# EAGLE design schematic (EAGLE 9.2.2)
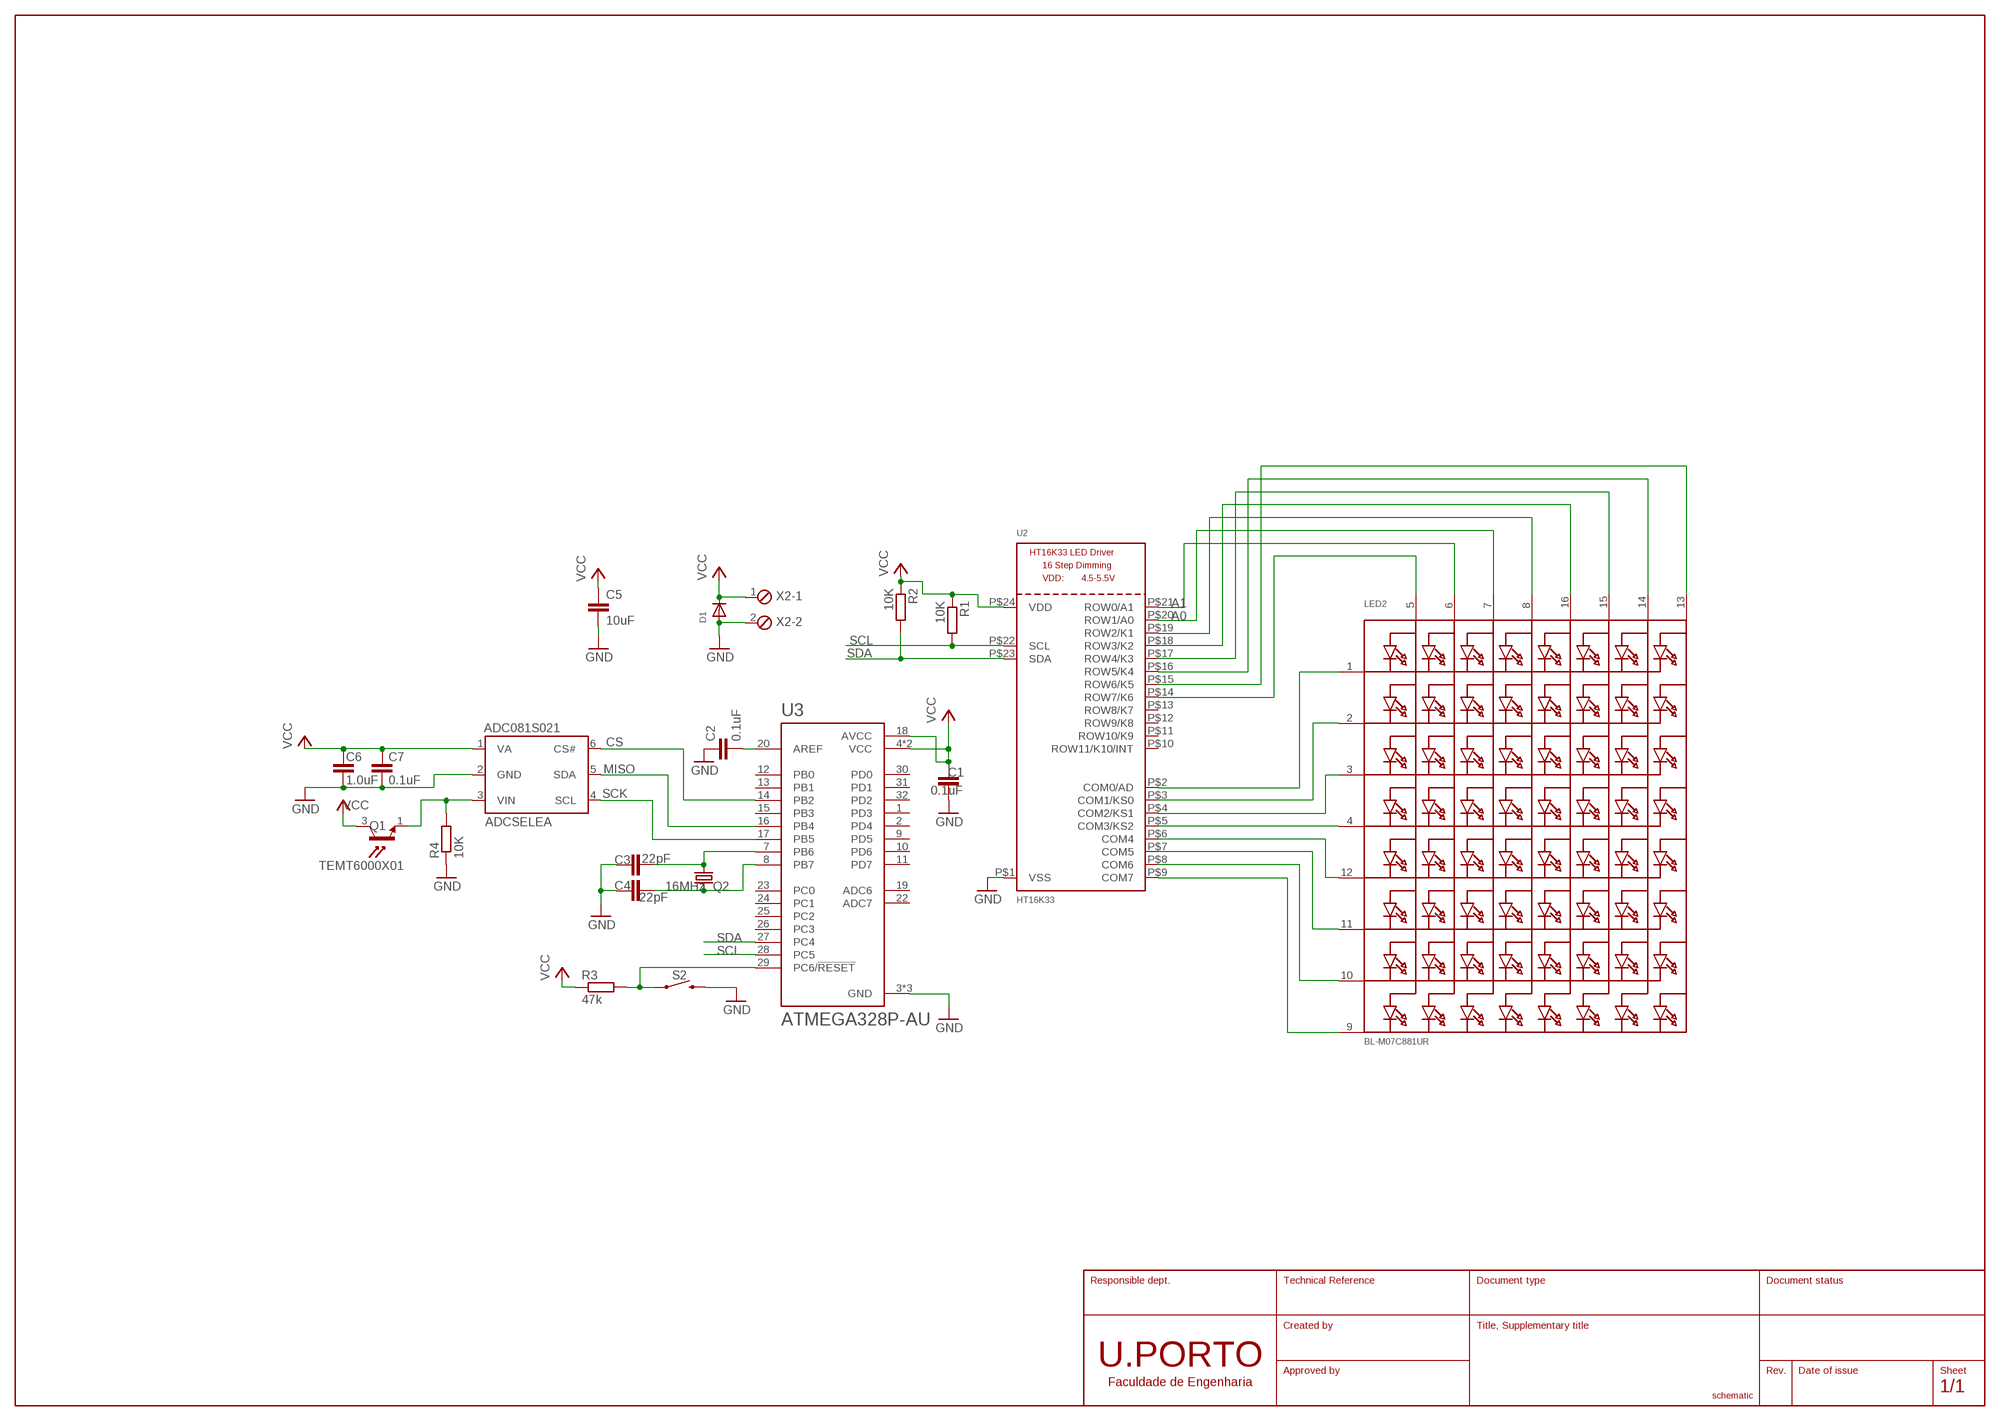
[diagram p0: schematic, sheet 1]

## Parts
ADC081S021  ADCSELEA  [SOT23]
C1  0.1uF  0.1UF-0402-16V-10%  [0402]
C2  0.1uF  0.1UF-0402-16V-10%  [0402]
C3  22pF  22PF-0603-50V-5%  [0603]
C4  22pF  22PF-0603-50V-5%  [0603]
C5  10uF  10UF-0603-6.3V-20%  [0603]
C6  1.0uF  1.0UF-0402-16V-10%  [0402]
C7  0.1uF  0.1UF-0402-16V-10%  [0402]
D1  DIODESOD-323F  [SOD-323F]
LED2  BL-M07C881UR  DISP_SEGMENT_8X8_ROWCATHODE  [SEGMENT_BL-M07C881UR]
Q1  TEMT6000X01  [TRANS_TEMT6000X01]
Q2  16MHz  CRYSTALCTS406  [CTS406]
R1  10K  R-EU_M0805  [M0805]
R2  10K  R-EU_M0805  [M0805]
R3  47k  R-EU_M0805  [M0805]
R4  10K  R-EU_M0805  [M0805]
S2  MOMENTARY-SWITCH-SPST-SMD-6.0X3.5MM  [TACTILE_SWITCH_SMD_6.0X3.5MM]
U2  HT16K33  HT16K33_SOP24  [SOP24_300MIL]
U3  ATMEGA328P-AU  [QFP80P900X900X120-32N]
X2  MPT2  [2POL254]

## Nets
A0 [LEDS]: LED2.7(A3) U2.P$20(ROW1/A0)
A1 [LEDS]: LED2.6(A2) U2.P$21(ROW0/A1)
CS [OTHER]: ADC081S021.6(CS#) U3.14(PB2)
GND [GND]: ADC081S021.2(GND) C1.1 C2.1 C3.1 C4.1 C5.2 C6.2 C7.2 D1.A R4.1 S2.2 U2.P$1(VSS) U3.3(GND) U3.5(GND) U3.21(GND) X2.2
MISO [OTHER]: ADC081S021.5(SDA) U3.16(PB4)
N$1 [OTHER]: C3.2 Q2.1 U3.7(PB6)
N$2 [OTHER]: C4.2 Q2.3 U3.8(PB7)
N$3 [OTHER]: C2.2 U3.20(AREF)
N$6 [LEDS]: LED2.9(K8) U2.P$9(COM7)
N$7 [LEDS]: LED2.10(K7) U2.P$8(COM6)
N$8 [LEDS]: LED2.11(K6) U2.P$7(COM5)
N$9 [LEDS]: LED2.12(K5) U2.P$6(COM4)
N$10 [LEDS]: LED2.4(K4) U2.P$5(COM3/KS2)
N$11 [LEDS]: LED2.3(K3) U2.P$4(COM2/KS1)
N$12 [LEDS]: LED2.2(K2) U2.P$3(COM1/KS0)
N$13 [LEDS]: LED2.1(K1) U2.P$2(COM0/AD)
N$14 [LEDS]: LED2.8(A4) U2.P$19(ROW2/K1)
N$15 [LEDS]: LED2.16(A5) U2.P$18(ROW3/K2)
N$16 [LEDS]: LED2.15(A6) U2.P$17(ROW4/K3)
N$17 [OTHER]: ADC081S021.3(VIN) Q1.1(E) R4.2
N$19 [LEDS]: LED2.5(A1) U2.P$14(ROW7/K6)
N$34 [OTHER]: R3.2 S2.1 U3.29(PC6/!RESET)
SCK [OTHER]: ADC081S021.4(SCL) U3.17(PB5)
SCL [OTHER]: R1.2 U2.P$22(SCL) U3.28(PC5)
SDA [OTHER]: R2.2 U2.P$23(SDA) U3.27(PC4)
SEG_F [LEDS]: LED2.14(A7) U2.P$16(ROW5/K4)
SEG_G [LEDS]: LED2.13(A8) U2.P$15(ROW6/K5)
VCC: ADC081S021.1(VA) C1.2 C5.1 C6.1 C7.1 D1.C Q1.3(C) R1.1 R2.1 R3.1 U2.P$24(VDD) U3.4(VCC) U3.6(VCC) U3.18(AVCC) X2.1
Unconnected: U2.P$10(ROW11/K10/INT) U2.P$11(ROW10/K9) U2.P$12(ROW9/K8) U2.P$13(ROW8/K7) U3.1(PD3) U3.2(PD4) U3.9(PD5) U3.10(PD6) U3.11(PD7) U3.12(PB0) U3.13(PB1) U3.15(PB3) U3.19(ADC6) U3.22(ADC7) U3.23(PC0) U3.24(PC1) U3.25(PC2) U3.26(PC3) U3.30(PD0) U3.31(PD1) U3.32(PD2)

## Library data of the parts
ADC081S021 = pmodals:ADCSELE
C1 C2 C7 = SparkFun-Capacitors:0.1UF: 0.1µF ceramic capacitors; PROD_ID: CAP-12416
C3 C4 = SparkFun-Capacitors:22PF: 22pF ceramic capacitors; PROD_ID: CAP-07876
C5 = SparkFun-Capacitors:10UF: 10.0µF ceramic capacitors; PROD_ID: CAP-11015
C6 = SparkFun-Capacitors:1.0UF: 1µF ceramic capacitors; PROD_ID: CAP-12417
D1 = adafruit:DIODE: Diode
LED2 = microbuilder:DISP_SEGMENT_8X8_ROWCATHODE: 8x8 LED Segment Displays: Row = Cathode 0.7" Red 8X8 Matrix, 1.9mm Round LEDs - BL-M07C881UR 1.2" Red 8x8 Matrix, 3.0mm Round LEDs - BL-M12A881UR 1.2" Red 8x8 Matrix, 3.0mm Square LEDs - BL-M12A883
Q1 = TEMT6000X01:TEMT6000X01: Ambient Light Sensor Phototransistor Chip Silicon 570nm Automotive 3-Pin SMD T/R; AVAILABILITY: Unavailable; DESCRIPTION: Ambient Light Sensor Phototransistor Chip Silicon 570nm Automotive 3-Pin SMD T/R; MF: Vishay Semiconductor; MP: TEMT6000X01; PACKAGE: 1206 Vishay; PRICE: None
Q2 = adafruit:CRYSTAL: CRYSTAL; OC_FARNELL: unknown; OC_NEWARK: unknown
R1-R4 = rcl:R-EU_: RESISTOR, European symbol; SPICEPREFIX: R
S2 = SparkFun-Switches:MOMENTARY-SWITCH-SPST: Momentary Switch (Pushbutton) - SPST; PROD_ID: SWCH-00815; SF_SKU: COM-08229
U2 = microbuilder:HT16K33_SOP24
U3 = ATMEGA328P-AU:ATMEGA328P-AU: ATmega Series 20 MHz 32 KB Flash 2 KB SRAM 8-Bit Microcontroller - TQFP-32; AVAILABILITY: Unavailable; DESCRIPTION: Microcontroller Mcu, 8 Bit, Atmega, 20mhz, Tqfp-32; MF: Microchip; MP: ATMEGA328P-AU; PACKAGE: TQFP-32 Microchip; PRICE: None
X2 = con-phoenix-254:MPT2: PHOENIX CONNECTOR; OC_FARNELL: unknown; OC_NEWARK: unknown

## Module ADC081S021
Ports: SDA(io) SCL(io) CS#(io) VA(io) GND(io) VIN(io)

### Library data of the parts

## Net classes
0 VCC: width 0.254 mm, clearance 0.203 mm
1 GND: width 0.254 mm, clearance 0.203 mm
2 OTHER: width 0.254 mm, clearance 0.203 mm
3 LEDS: width 0.254 mm, clearance 0.203 mm

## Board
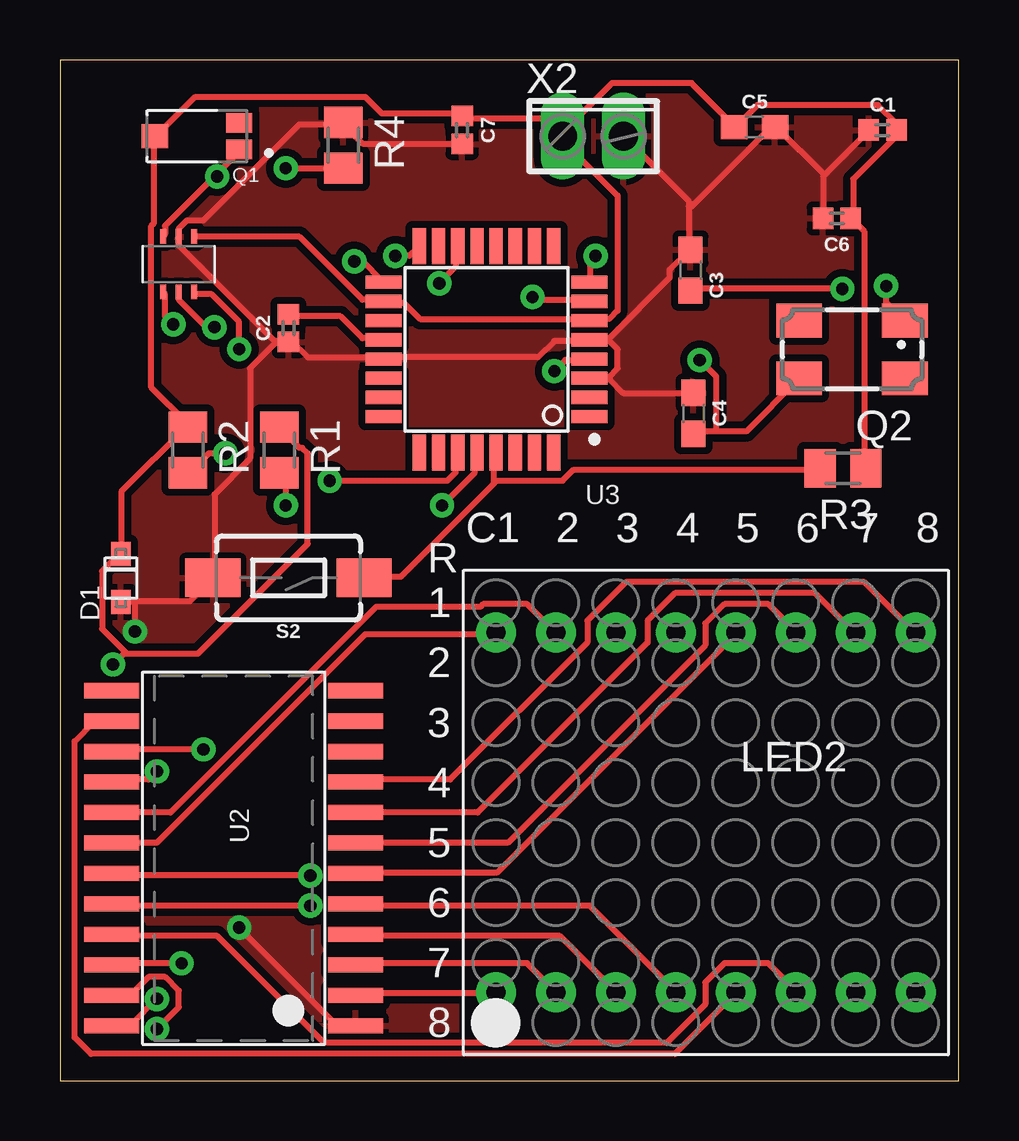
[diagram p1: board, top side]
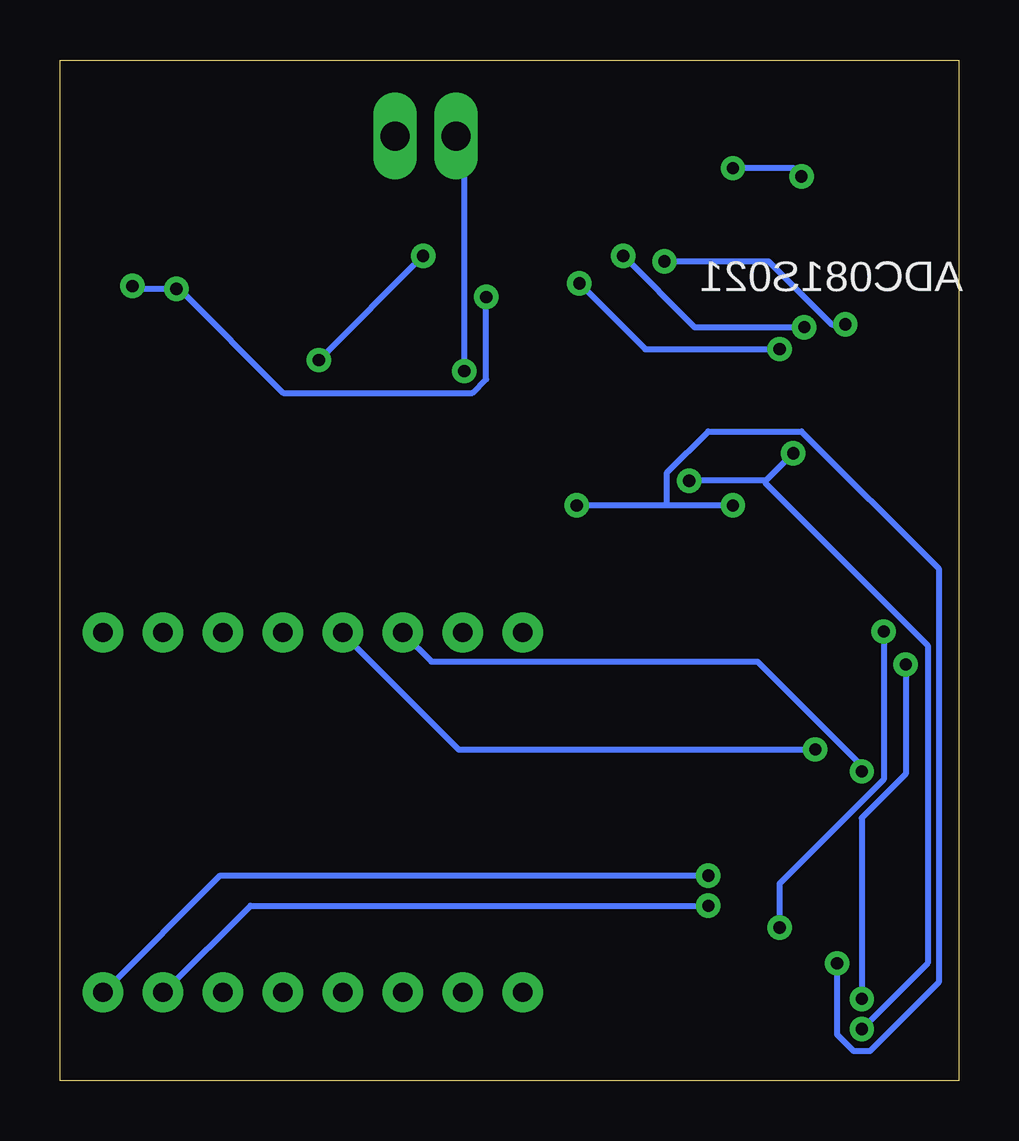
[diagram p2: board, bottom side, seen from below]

Size 37.47 x 42.55 mm. Coordinates in mm from the lower left corner, seen from the top.
Outline: 0,0 37.47,0 37.47,42.55 0,42.55 0,0
Copper layers (1*16): Top 0.035mm / dielectric 1.5mm / Bottom 0.035mm
Design rules "SparkFun": minimum track width 8mil, minimum drill 20mil, track to track 8mil, track to pad 8mil, pad to pad 8mil, via to via 8mil, smd to smd 8mil, copper to edge 10mil, drill to drill 8mil, minimum pad ring 12mil, minimum via ring 10mil, stop-mask expansion 4mil, vias tented up to drill 25mil, thermal gap 10mil

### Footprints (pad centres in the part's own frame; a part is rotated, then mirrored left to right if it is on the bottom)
SOT23 = smd 0.25 x 0.6: 1 -0.65,-1.15; 2 0,-1.15; 3 0.65,-1.15; 4 0.65,1.15; 5 0,1.15; 6 -0.65,1.15
0402 = smd 0.85 x 0.9: 1 -0.58,0; 2 0.58,0
0603 = smd 1.1 x 1: 1 -0.85,0; 2 0.85,0
SOD-323F = smd 1 x 0.8: A -1,0; C 1,0
SEGMENT_BL-M07C881UR = drill 0.8 pad 1.676: 1 -8.75,-7.5; 2 -6.25,-7.5; 3 -3.75,-7.5; 4 -1.25,-7.5; 5 1.25,-7.5; 6 3.75,-7.5; 7 6.25,-7.5; 8 8.75,-7.5; 9 8.75,7.5; 10 6.25,7.5; 11 3.75,7.5; 12 1.25,7.5; 13 -1.25,7.5; 14 -3.75,7.5; 15 -6.25,7.5; 16 -8.75,7.5
TRANS_TEMT6000X01 = smd 1.1 x 0.8: 1 -1.755,0.55; 2 -1.755,-0.55 | smd 1.1 x 1: 3 1.755,0
CTS406 = smd 1.9 x 1.4: 1 -2.2,-1.2; 2 2.2,-1.2; 3 2.2,1.2; 4 -2.2,1.2
M0805 = smd 1.3 x 1.6: 1 -0.95,0; 2 0.95,0
TACTILE_SWITCH_SMD_6.0X3.5MM = smd 2.3 x 1.6: 1 -3.15,0; 2 3.15,0
SOP24_300MIL = smd 0.635 x 2.286: P$1 -6.985,-5.08; P$2 -5.715,-5.08; P$3 -4.445,-5.08; P$4 -3.175,-5.08; P$5 -1.905,-5.08; P$6 -0.635,-5.08; P$7 0.635,-5.08; P$8 1.905,-5.08; P$9 3.175,-5.08; P$10 4.445,-5.08; P$11 5.715,-5.08; P$12 6.985,-5.08; P$13 6.985,5.08; P$14 5.715,5.08; P$15 4.445,5.08; P$16 3.175,5.08; P$17 1.905,5.08; P$18 0.635,5.08; P$19 -0.635,5.08; P$20 -1.905,5.08; P$21 -3.175,5.08; P$22 -4.445,5.08; P$23 -5.715,5.08; P$24 -6.985,5.08
QFP80P900X900X120-32N = smd 1.5 x 0.55: 1 -4.3,2.8; 2 -4.3,2; 3 -4.3,1.2; 4 -4.3,0.4; 5 -4.3,-0.4; 6 -4.3,-1.2; 7 -4.3,-2; 8 -4.3,-2.8; 17 4.3,-2.8; 18 4.3,-2; 19 4.3,-1.2; 20 4.3,-0.4; 21 4.3,0.4; 22 4.3,1.2; 23 4.3,2; 24 4.3,2.8 | smd 0.55 x 1.5: 9 -2.8,-4.3; 10 -2,-4.3; 11 -1.2,-4.3; 12 -0.4,-4.3; 13 0.4,-4.3; 14 1.2,-4.3; 15 2,-4.3; 16 2.8,-4.3; 25 2.8,4.3; 26 2,4.3; 27 1.2,4.3; 28 0.4,4.3; 29 -0.4,4.3; 30 -1.2,4.3; 31 -2,4.3; 32 -2.8,4.3
2POL254 = drill 1.2 long: 1 -1.27,0; 2 1.27,0

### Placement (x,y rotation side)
ADC081S021  4.95,34.04 180 top
C1  34.29,39.62 0 top
C2  9.53,31.37 90 top
C3  26.29,33.78 270 top
C4  26.42,27.81 270 top
C5  28.96,39.75 0 top
C6  32.38,35.94 180 top
C7  16.76,39.62 270 top
D1  2.54,20.95 90 top
LED2  26.92,11.18 0 top
Q1  5.71,39.37 180 top
Q2  33.02,30.48 180 top
R1  9.14,26.29 270 top
R2  5.33,26.29 270 top
R3  32.64,25.53 180 top
R4  11.81,38.99 270 top
S2  9.53,20.95 180 top
U2  7.24,9.27 90 top
U3  17.78,30.48 180 top
X2  22.23,39.37 0 top

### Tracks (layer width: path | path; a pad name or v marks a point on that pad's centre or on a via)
A0  (via drill 0.51)
  Top 0.254: v10.44,7.29 2.21,7.29 U2.P$20
  Bottom 0.254: v10.44,7.29 29.53,7.29 33.07,3.75 LED2.7
A1
  Top 0.254: U2.P$21 2.21,6.03 6.55,6.03 11.01,1.57 25.3,1.57 26.9,3.17 26.9,4.09 27.7,4.89 29.53,4.89 30.67,3.75 LED2.6
CS  (via drill 0.51)
  Top 0.254: v7.47,30.49 7.47,31.64 6.33,32.78 5.64,32.78 ADC081S021.6 | v15.81,33.24 16.5,33.92 16.5,34.72 U3.14
  Bottom 0.254: v7.47,30.49 13.07,30.49 v15.81,33.24
GND  (via drill 0.51)
  Top 0.254: 3.12,19.98 5.41,19.98 6.33,20.89 S2.2 6.44,21.01 6.44,24.43 7.92,25.92 7.92,29.69 8.95,30.72 8.95,30.84 | 3.12,19.98 2.55,19.98 D1.A | v7.47,6.38 11.47,2.38 12.27,2.38 U2.P$1 | 3.12,19.98 v3.12,18.72 | C7.2 16.73,39.06 12.61,39.06 11.81,39.87 R4.1 11.7,39.87 9.98,39.87 5.98,35.87 5.3,35.87 4.95,35.52 ADC081S021.2 4.95,34.84 8.95,30.84 | 8.95,30.84 9.53,30.84 C2.1 9.64,30.84 10.32,30.15 13.41,30.15 U3.21 13.53,30.15 19.93,30.15 20.61,30.84 21.98,30.84 U3.5 22.1,30.84 22.9,30.84 | 31.81,37.69 31.81,35.98 C6.2 | 31.81,37.69 33.64,39.52 C1.1 | 31.81,37.69 31.81,37.81 29.87,39.75 C5.2 29.76,39.64 29.53,39.64 26.33,36.44 26.21,36.44 | 22.9,29.23 23.47,28.66 26.33,28.66 C4.1 | 22.9,29.23 22.1,29.23 U3.3 | 22.9,30.84 23.24,30.49 23.24,29.69 22.9,29.35 22.9,29.23 | 26.21,36.44 26.21,36.66 23.58,39.29 X2.2 | 26.21,36.44 26.21,34.72 C3.1 26.21,34.61 25.41,33.81 25.41,33.47 22.9,30.95 22.9,30.84
  Bottom 0.254: v7.47,6.38 7.47,8.2 3.12,12.55 v3.12,18.72
  pour Top (isolate 0.305): 16.51,0 0,0 0,42.55 37.47,42.55 37.47,21.59 16.51,21.59
MISO  (via drill 0.51)
  Top 0.254: ADC081S021.5 4.95,32.55 6.1,31.41 v6.44,31.41 | v13.98,34.38 14.55,34.38 14.9,34.72 U3.16
  Bottom 0.254: v6.44,31.41 11.01,31.41 v13.98,34.38
N$1  (via drill 0.51)
  Top 0.254: v32.61,33.01 26.33,33.01 C3.2 | v34.44,33.12 34.44,32.44 35.13,31.75 Q2.1 | v19.7,32.66 19.81,32.55 21.98,32.55 U3.7
  Bottom 0.254: v34.44,33.12 34.33,33.01 v32.61,33.01 32.5,33.01 28.16,28.66 20.27,28.66 19.7,29.23 v19.7,32.66
N$2  (via drill 0.51)
  Top 0.254: 27.36,27.06 28.61,27.06 30.79,29.23 Q2.3 | 27.36,27.06 26.44,27.06 C4.2 | v22.33,34.38 22.1,34.15 22.1,33.35 U3.8 | v26.67,30.04 27.36,29.35 27.36,27.06
  Bottom 0.254: v26.67,30.04 v22.33,34.38
N$3
  Top 0.254: C2.2 9.53,31.86 11.7,31.86 12.61,30.95 13.41,30.95 U3.20
N$6
  Top 0.254: U2.P$9 12.38,12.55 16.27,12.55 21.98,18.26 21.98,19.18 23.58,20.78 33.53,20.78 35.59,18.72 LED2.9
N$7
  Top 0.254: U2.P$8 17.41,11.18 24.5,18.26 24.5,19.18 25.64,20.32 31.47,20.32 33.07,18.72 LED2.10
N$8
  Top 0.254: U2.P$7 12.38,9.92 18.67,9.92 26.9,18.15 26.9,19.06 27.7,19.86 29.53,19.86 30.67,18.72 LED2.11
N$9
  Top 0.254: U2.P$6 12.38,8.66 18.21,8.66 28.16,18.61 LED2.12
N$10
  Top 0.254: U2.P$5 12.38,7.29 22.1,7.29 25.64,3.75 LED2.4
N$11
  Top 0.254: U2.P$4 12.38,6.03 20.84,6.03 23.13,3.75 LED2.3
N$12
  Top 0.254: U2.P$3 12.38,4.89 19.47,4.89 20.61,3.75 LED2.2
N$13
  Top 0.254: U2.P$2 12.38,3.63 18.1,3.63 LED2.1
N$14  (via drill 0.51)
  Top 0.254: v10.44,8.55 2.21,8.55 U2.P$19
  Bottom 0.254: v10.44,8.55 30.79,8.55 35.59,3.75 LED2.8
N$15
  Top 0.254: U2.P$18 2.21,9.92 4.04,9.92 12.72,18.61 18.1,18.61 LED2.16
N$16
  Top 0.254: U2.P$17 4.61,11.18 13.18,19.75 17.53,19.75 17.64,19.86 19.47,19.86 20.61,18.72 LED2.15
N$17  (via drill 0.51)
  Top 0.254: 6.5,37.75 7.47,38.72 Q1.1 | 6.5,37.75 4.38,35.64 4.38,35.29 ADC081S021.3 | v9.41,38.04 R4.2 | v6.55,37.69 6.5,37.75
  Bottom 0.254: v9.41,38.04 6.9,38.04 v6.55,37.69
N$19
  Top 0.254: U2.P$14 2.1,14.95 1.41,14.95 0.61,14.15 0.61,1.8 1.29,1.12 25.64,1.12 28.16,3.63 LED2.5
N$34
  Top 0.254: 18.1,25.01 18.1,24.89 14.21,21.01 12.72,21.01 S2.1 | 18.1,25.01 18.1,26.15 U3.29 | 18.1,25.01 20.95,25.01 21.41,25.46 31.59,25.46 R3.2
SCK  (via drill 0.51)
  Top 0.254: v4.72,31.52 4.38,31.86 4.38,32.78 ADC081S021.4 | v12.27,34.15 12.61,34.15 13.41,33.35 U3.17
  Bottom 0.254: v4.72,31.52 5.3,31.52 7.92,34.15 v12.27,34.15
SCL  (via drill 0.51)
  Top 0.254: v15.93,23.98 17.3,25.35 17.3,26.15 U3.28 | v9.41,23.98 9.41,25.01 9.18,25.23 R1.2 | v5.07,4.89 2.21,4.89 U2.P$22
  Bottom 0.254: v9.41,23.98 12.15,23.98 | 12.15,23.98 v15.93,23.98 | v5.07,4.89 5.07,1.92 4.38,1.23 3.7,1.23 0.84,4.09 0.84,21.35 6.55,27.06 10.44,27.06 12.15,25.35 12.15,23.98
SDA  (via drill 0.51)
  Top 0.254: v11.24,25.01 16.15,25.01 16.5,25.35 16.5,26.15 U3.27 | v6.9,26.15 6.21,26.15 5.41,25.35 R2.2 | v4.04,2.15 4.95,3.06 4.95,3.75 4.38,4.32 3.7,4.32 3.01,3.63 2.21,3.63 U2.P$23
  Bottom 0.254: 8.04,25.01 v11.24,25.01 | v6.9,26.15 8.04,25.01 | v4.04,2.15 1.29,4.89 1.29,18.15 8.04,24.89 8.04,25.01
SEG_F  (via drill 0.51)
  Top 0.254: v4.04,12.89 3.7,12.55 2.21,12.55 U2.P$16
  Bottom 0.254: v4.04,12.89 4.04,13.12 8.38,17.46 21.98,17.46 23.13,18.61 LED2.14
SEG_G  (via drill 0.51)
  Top 0.254: v5.98,13.8 2.21,13.8 U2.P$15
  Bottom 0.254: v5.98,13.8 20.84,13.8 25.64,18.61 LED2.13
VCC  (via drill 0.51)
  Top 0.254: ADC081S021.1 5.64,35.18 9.98,35.18 12.61,32.55 13.41,32.55 U3.18 13.53,32.44 14.33,32.44 15.01,31.75 21.98,31.75 U3.6 22.1,31.75 22.9,31.75 23.24,32.09 23.24,36.89 20.95,39.18 X2.1 | X2.1 20.95,39.41 20.27,40.09 16.84,40.09 C7.1 16.73,40.32 13.41,40.32 12.72,41.01 5.64,41.01 4.04,39.41 Q1.3 3.92,39.29 3.92,35.75 3.81,35.64 3.81,28.89 5.3,27.41 R2.1 5.3,27.29 2.55,24.55 2.55,22.04 D1.C 2.44,21.92 1.75,21.23 1.75,18.83 2.78,17.8 | v20.61,29.58 21.07,30.04 21.98,30.04 U3.4 | R3.1 33.53,25.58 33.53,35.41 33.07,35.87 C6.1 33.07,35.98 33.07,37.58 34.78,39.29 34.78,39.52 C1.2 34.9,39.75 34.9,39.87 34.1,40.66 29.07,40.66 28.16,39.75 C5.1 28.04,39.87 26.33,41.58 23.01,41.58 20.95,39.52 X2.1 | 2.78,17.8 5.75,17.8 10.32,22.38 10.32,26.15 10.1,26.38 9.98,26.38 9.18,27.18 R1.1 | v4.04,3.4 3.01,2.38 2.21,2.38 U2.P$24 | v2.21,17.35 2.67,17.8 2.78,17.8
  Bottom 0.254: v20.61,29.58 20.61,38.95 20.95,39.29 X2.1 | v4.04,3.4 4.04,10.95 2.21,12.78 v2.21,17.35

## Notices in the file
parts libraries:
SparkFun-Capacitors: Licensing: Creative Commons ShareAlike 4.0 International - https://creativecommons.org/licenses/by-sa/4.0
